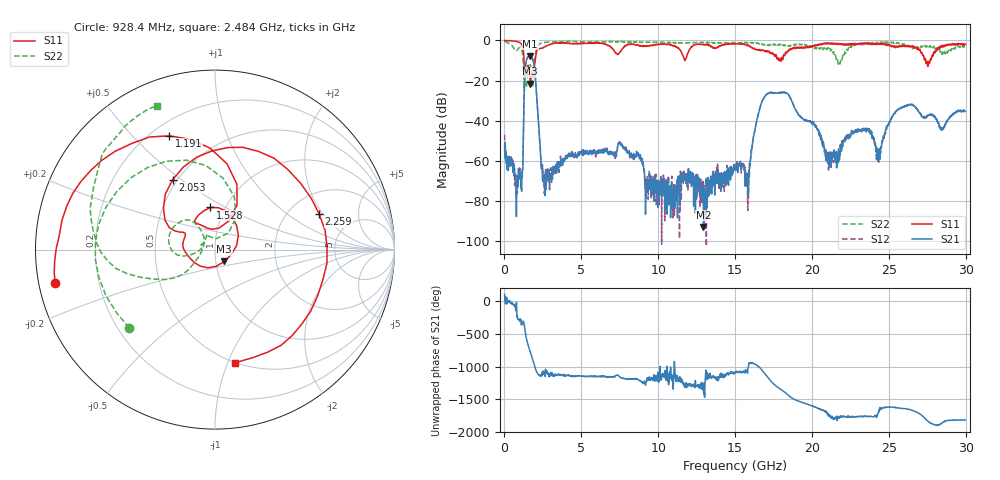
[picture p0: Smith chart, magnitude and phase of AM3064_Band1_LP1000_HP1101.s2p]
# Hz S DB R 50.0
!freq dBS11 angS11 dBS21 angS21 dBS12 angS12 dBS22 angS22
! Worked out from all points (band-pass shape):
!   1600 points, 10 MHz to 29.98 GHz, reference 50 ohm
!   highest |S21| = -7.82 dB at 1.678 GHz (marker M1); lowest = -93.0 dB at 12.94 GHz (marker M2)
!   |S21| within 3 dB of the highest: 1.405 GHz to 1.891 GHz (486.5 MHz wide, 29.5 % of centre)
!   lowest |S11| = -21.5 dB at 1.678 GHz (marker M3), VSWR 1.18, Z = 55 - j7.32 ohm
!   |S11| at or under -10 dB: 1.277 GHz to 1.993 GHz (716.4 MHz wide, 43.8 % of centre); 11.72193 GHz to 11.74409 GHz (22.16 MHz wide, 0.189 % of centre); 27.4 GHz to 27.68 GHz (282.2 MHz wide, 1.02 % of centre)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
!   |S22| runs from -24.3 to -0.3 dB; largest |S21 - S12| = 0.0049
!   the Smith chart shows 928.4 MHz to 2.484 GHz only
!   S11 on the Smith chart (normalised r, x): 928.4 MHz: 0.05, -0.10; 1.191 GHz: 0.27, +0.64; 1.528 GHz: 0.85, +0.42; 2.053 GHz: 0.47, +0.46; 2.259 GHz: 2.90, +1.84; 2.484 GHz: 0.50, -1.06
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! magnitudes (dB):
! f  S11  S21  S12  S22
! 10 MHz  0.0  -52.4  -47.0  -0.3
! 928.4 MHz  -0.8  -68.4  -67.9  -3.8
! 1.191 GHz  -3.3  -64.4  -63.1  -8.0
! 1.528 GHz  -12.5  -8.3  -8.2  -13.5
! 1.678 GHz  -21.5  -7.8  -7.8  -12.1
! 2.053 GHz  -6.8  -23.0  -22.9  -5.0
! 2.259 GHz  -4.2  -46.0  -45.9  -1.9
! 2.484 GHz  -3.9  -70.3  -62.3  -1.3
! 5.015 GHz  -1.4  -55.3  -56.3  -0.6
! 7.564 GHz  -5.5  -51.6  -51.0  -0.5
! 10 GHz  -2.0  -70.7  -69.7  -0.9
! 12.94 GHz  -2.1  -93.0  -75.3  -1.0
! 15 GHz  -1.7  -63.5  -61.8  -1.4
! 15.83 GHz  -2.7  -68.9  -84.7  -1.4
! 16.45 GHz  -4.7  -38.8  -38.8  -1.5
! 17.14 GHz  -5.7  -26.4  -26.3  -2.5
! 19.99 GHz  -3.4  -40.5  -40.8  -3.1
! 21.15 GHz  -1.3  -59.1  -59.8  -4.0
! 23.5 GHz  -1.6  -44.1  -44.5  -1.7
! 24.32 GHz  -1.9  -54.8  -57.8  -0.9
! 25 GHz  -2.0  -41.8  -41.2  -1.1
! 29.98 GHz  -1.8  -35.3  -35.1  -3.1
